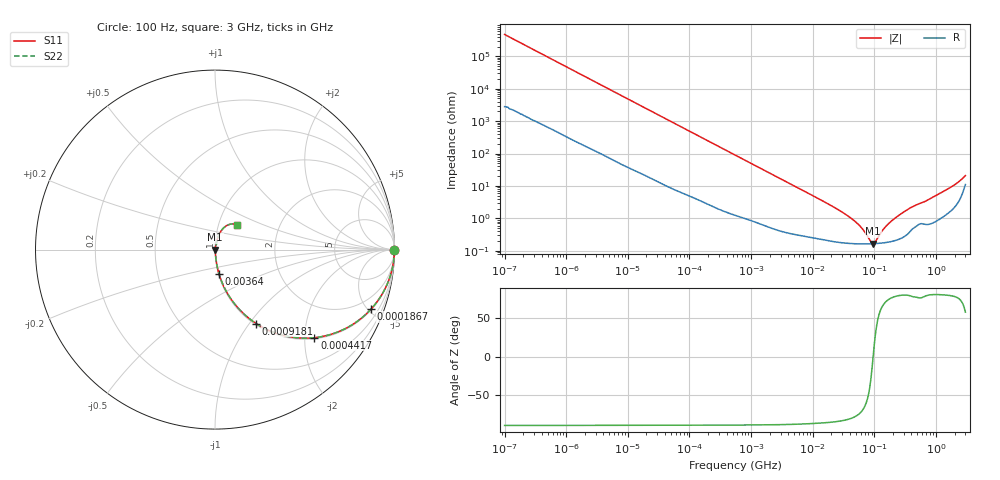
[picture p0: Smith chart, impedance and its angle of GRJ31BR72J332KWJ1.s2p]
!Murata Part Number: GRJ31BR72J332KWJ1
!These Parameters are Measured in Series Mode Connection
!Data Generated on Jun 19, 2026
!  o--ll--o
!Port1  Port2
!  o------o
!Operation Temp=25[degC], DC Bias Voltage=0[V]
!Freq. Start=100[Hz] Stop=3[GHz] 401[Steps]
# Hz S RI R 50
!Freq.(Hz) S11(Real) S11(Imag) S21(Real) S21(Imag) S12(Real) S12(Imag) S22(Real) S22(Imag)
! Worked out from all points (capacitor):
!   401 points, 100 Hz to 3 GHz, reference 50 ohm
!   read as one part in series: C = 3.37 nF near 109 Hz
!   lowest |Z| = 165 mohm at 95.87 MHz (marker M1)
!   series resonance near 95.55 MHz, so ESL is about 820 pH
!   S11 on the Smith chart (normalised r, x): 100 Hz: open; 186.7 kHz: 1.06, -5.25; 441.7 kHz: 1.03, -2.23; 918.1 kHz: 1.02, -1.08; 3.64 MHz: 1.01, -0.28; 3 GHz: 1.22, +0.35
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100  1 -0.000212  1.3e-06 0.000212  1.3e-06 0.000212  1 -0.000212
1788  1 -0.00374  4.06e-05 0.00374  4.06e-05 0.00374  1 -0.00374
31977  0.9951 -0.0656  0.00488 0.0656  0.00488 0.0656  0.9951 -0.0656
93790  0.9626 -0.1848  0.0374 0.1848  0.0374 0.1848  0.9626 -0.1848
186741  0.8704 -0.3304  0.1296 0.3304  0.1296 0.3304  0.8704 -0.3304
441669  0.5535 -0.4907  0.4465 0.4907  0.4465 0.4907  0.5535 -0.4907
547723  0.4484 -0.4905  0.5516 0.4905  0.5516 0.4905  0.4484 -0.4905
918067  0.2293 -0.4121  0.7707 0.4121  0.7707 0.4121  0.2293 -0.4121
1677156  0.0856 -0.2701  0.9144 0.2701  0.9144 0.2701  0.0856 -0.2701
3639519  0.022 -0.1341  0.978 0.1341  0.978 0.1341  0.022 -0.1341
9794414  0.00513 -0.0509  0.9949 0.0509  0.9949 0.0509  0.00513 -0.0509
2.52476e7  0.00219 -0.0189  0.9978 0.0189  0.9978 0.0189  0.00219 -0.0189
4.418008e7  0.00174 -0.00918  0.9983 0.00918  0.9983 0.00918  0.00174 -0.00918
5.9714e7  0.00165 -0.00527  0.9983 0.00527  0.9983 0.00527  0.00165 -0.00527
8.79653e7  0.00164 -0.000896  0.9984 0.000896  0.9984 0.000896  0.00164 -0.000896
9.587315e7  0.00165 3.68e-05  0.9984 -3.68e-05  0.9984 -3.68e-05  0.00165 3.68e-05
1.044919e8  0.00166 0.00097  0.9983 -0.00097  0.9983 -0.00097  0.00166 0.00097
1.352818e8  0.00175 0.00385  0.9983 -0.00385  0.9983 -0.00385  0.00175 0.00385
1.751444e8  0.00192 0.00699  0.9981 -0.00699  0.9981 -0.00699  0.00192 0.00699
3.640608e8  0.00395 0.0195  0.9961 -0.0195  0.9961 -0.0195  0.00395 0.0195
1.789813e9  0.0255 0.0891  0.9745 -0.0891  0.9745 -0.0891  0.0255 0.0891
3e9  0.1217 0.1398  0.8783 -0.1398  0.8783 -0.1398  0.1217 0.1398
